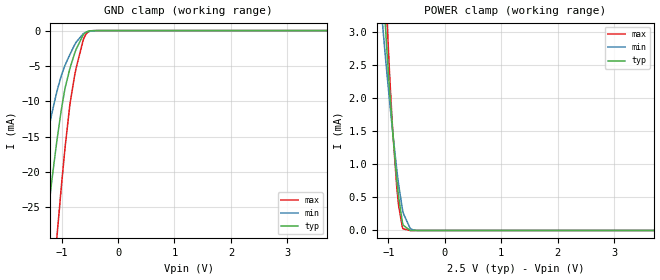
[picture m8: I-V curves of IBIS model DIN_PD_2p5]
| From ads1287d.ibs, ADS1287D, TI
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|   Model
[Model]   DIN_PD_2p5
Model_type   Input
Vinl = 0.75
Vinh = 1.75
|   typ   min   max
C_comp   2.168pF   1.862pF   2.430pF
[Voltage Range]   2.5   2.2   2.8
[Temperature Range]   27   125   -40
[Power Clamp Reference]   2.5   2.2   2.8
[GND Clamp Reference]   0   0   0
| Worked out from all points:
|   GND clamp passes 1 mA (typ) near -0.64 V on its own axis
|   POWER clamp passes 1 mA (typ) near -0.88 V on its own axis
[GND Clamp]
|   Voltage   I(typ)   I(min)   I(max)
-2.5V     -133.8mA   -86.37mA   -178.9mA
-1.607V   -54.39mA   -31.73mA   -82.87mA
-1.532V   -48.22mA   -27.84mA   -74.92mA
-1.353V   -34.08mA   -19.19mA   -56.08mA
-1.248V   -26.4mA    -14.68mA   -45.35mA
-1.075V   -15.13mA   -8.39mA    -28.53mA
-955mV    -8.886mA   -5.244mA   -17.96mA
-850mV    -5.305mA   -3.343mA   -10.35mA
-745mV    -2.705mA   -1.675mA   -5.407mA
-617.5mV  -603.1uA   -456.5uA   -1.351mA
-550mV    -160.9uA   -201.9uA   -347.2uA
5V        0A         0A         0A
[POWER Clamp]
|   Voltage   I(typ)   I(min)   I(max)
-2.5V     29.7mA     23.21mA    36.25mA
-1.097V   3.739mA    3.048mA    4.602mA
-1.06V    3.177mA    2.683mA    3.849mA
-1.038V   2.86mA     2.472mA    3.411mA
-1.022V   2.657mA    2.334mA    3.127mA
-925mV    1.497mA    1.486mA    1.514mA
-857.5mV  824.6uA    957.1uA    710uA
-820mV    507.9uA    695.7uA    375uA
-737.5mV  79.08uA    261.9uA    23.79uA
-617.5mV  980.7nA    34.48uA    42.61nA
-497.5mV  0A         1.632uA    0A
5V        0A         0A         0A
